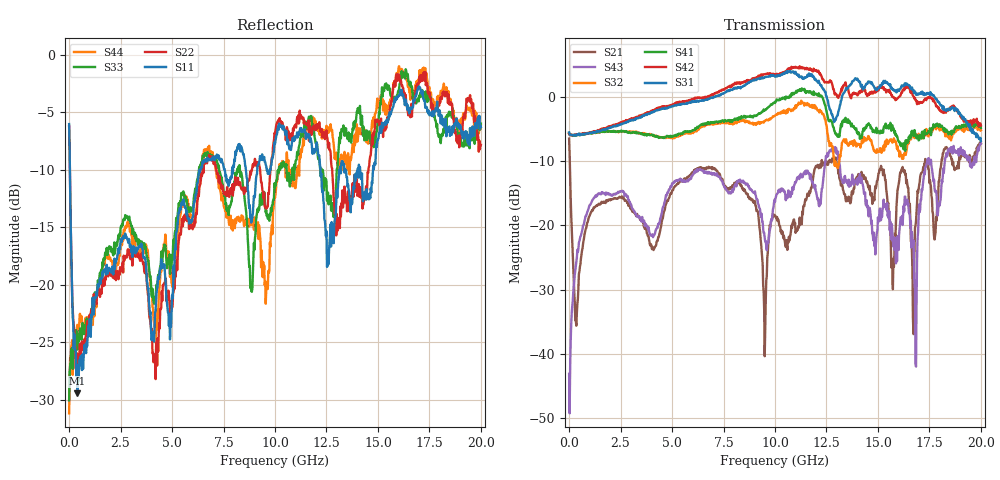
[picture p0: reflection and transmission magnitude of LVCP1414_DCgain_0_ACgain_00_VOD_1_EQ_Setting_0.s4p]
!Agilent Technologies,N5230A,MY46400459,A.07.50.48
!Agilent N5230A: A.07.50.48
!Date: Tuesday, April 17, 2012 18:25:30
!Correction: S11(Full 4 Port(1,2,3,4))
!S12(Full 4 Port(1,2,3,4))
!S13(Full 4 Port(1,2,3,4))
!S14(Full 4 Port(1,2,3,4))
!S21(Full 4 Port(1,2,3,4))
!S22(Full 4 Port(1,2,3,4))
!S23(Full 4 Port(1,2,3,4))
!S24(Full 4 Port(1,2,3,4))
!S31(Full 4 Port(1,2,3,4))
!S32(Full 4 Port(1,2,3,4))
!S33(Full 4 Port(1,2,3,4))
!S34(Full 4 Port(1,2,3,4))
!S41(Full 4 Port(1,2,3,4))
!S42(Full 4 Port(1,2,3,4))
!S43(Full 4 Port(1,2,3,4))
!S44(Full 4 Port(1,2,3,4))
!S4P File: Measurements: <S11,S12,S13,S14>,
!<S21,S22,S23,S24>,
!<S31,S32,S33,S34>,
!<S41,S42,S43,S44>:
# Hz S  dB  R 50
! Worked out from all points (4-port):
!   801 points, 300 kHz to 20 GHz, reference 50 ohm
!   strongest paths, dB at 300 kHz, 5 GHz, 10 GHz, 15 GHz, 20 GHz:
!     S31: -5.5, -1.4, 3.2, 1.3, -6.9
!     S42: -5.7, -1.2, 3.5, 1.5, -4.4
!     S41: -5.6, -6.1, -0.9, -5.2, -4.8
!     S32: -5.7, -6.4, -2.9, -8.5, -5.2
!     S43: -43.1, -13.5, -16.3, -18.7, -7.2
!     S21: -6.5, -14.5, -18.5, -12.6, -7.2
!   lowest |S11| = -29.4 dB at 400.3 MHz (marker M1), VSWR 1.07, Z = 53.2 + j1.4 ohm
!   |S11| at or under -10 dB: 37.53 MHz to 6.37 GHz (6.333 GHz wide, 198 % of centre); 12.21 GHz to 13.12 GHz (918.3 MHz wide, 7.25 % of centre); 14.14 GHz to 14.76 GHz (624.8 MHz wide, 4.32 % of centre)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
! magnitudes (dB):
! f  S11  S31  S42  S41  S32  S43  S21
! 300 kHz  -6.0  -5.5  -5.7  -5.6  -5.7  -43.1  -6.5
! 400.3 MHz  -29.4  -5.8  -5.8  -5.9  -5.8  -23.8  -32.2
! 10.08 GHz  -7.0  3.4  3.6  -0.4  -2.7  -15.2  -19.0
! 12.88 GHz  -14.8  -3.9  0.8  -5.2  -10.0  -8.2  -9.5
! 16.8 GHz  -3.8  0.8  -0.1  -5.5  -5.8  -29.9  -20.3
! 18.05 GHz  -6.0  -1.3  -2.2  -4.7  -4.6  -15.8  -11.0
! 20 GHz  -6.3  -6.9  -4.4  -4.8  -5.2  -7.2  -7.2
